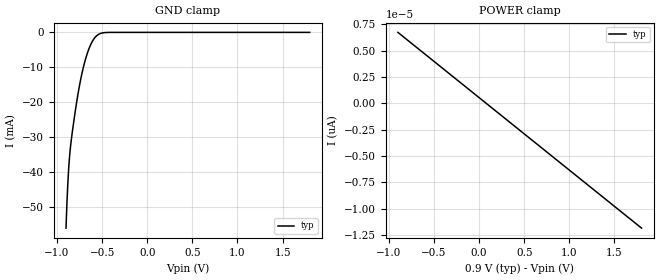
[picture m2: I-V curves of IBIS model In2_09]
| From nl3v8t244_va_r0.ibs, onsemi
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|//////////////////////////////////////////////////////////////////////////////
|//////////////////////////////////////////////////////////////////////////////
[Model]  In2_09
Model_type Input
Vinh =  0.81
Vinl =  0.09
|  variable   typ   min   max
C_comp   4.8pF   4.8pF   4.8pF
|//////////////////////////////////////////////////////////////////////////////
[Temperature Range]   25   125   -40
|//////////////////////////////////////////////////////////////////////////////
[Voltage Range]   0.90V   NA   NA
|//////////////////////////////////////////////////////////////////////////////
[POWER Clamp Reference] 0.90V   NA   NA
|//////////////////////////////////////////////////////////////////////////////
[GND Clamp Reference]   0V   NA   NA
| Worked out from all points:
|   GND clamp passes 1 mA (typ) near -0.56 V on its own axis
|//////////////////////////////////////////////////////////////////////////////
[GND Clamp]
|   Voltage   I(typ)   I(min)   I(max)
-900mV    -55.97mA   NA         NA
-890mV    -49.01mA   NA         NA
-880mV    -43.23mA   NA         NA
-860mV    -35.28mA   NA         NA
-830mV    -28.47mA   NA         NA
-780mV    -19.63mA   NA         NA
-730mV    -12.54mA   NA         NA
-680mV    -7.319mA   NA         NA
-620mV    -3.149mA   NA         NA
-560mV    -954.7uA   NA         NA
-420mV    -11.1uA    NA         NA
1.8V      6.738pA    NA         NA
|//////////////////////////////////////////////////////////////////////////////
[POWER Clamp]
|   Voltage   I(typ)   I(min)   I(max)
-900mV    6.738pA    NA         NA
0V        548.1fA    NA         NA
900mV     -5.642pA   NA         NA
1.8V      -11.83pA   NA         NA
